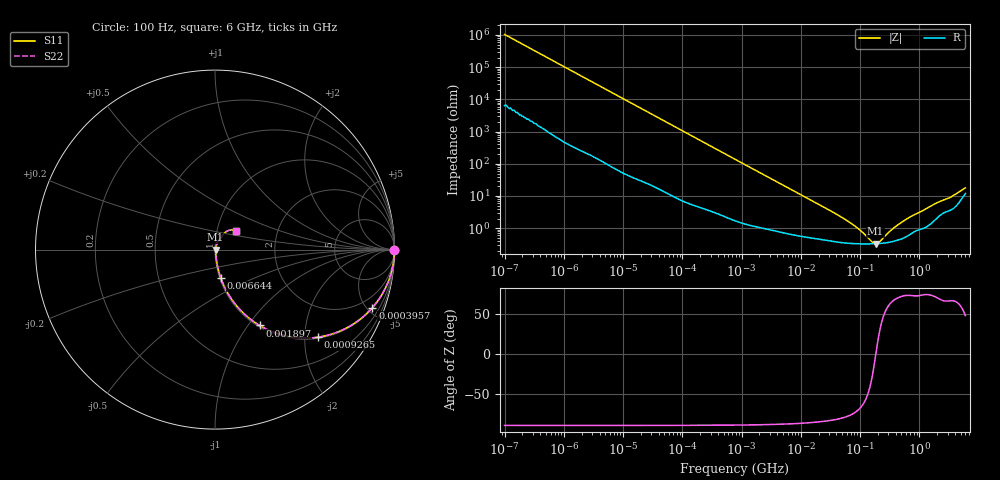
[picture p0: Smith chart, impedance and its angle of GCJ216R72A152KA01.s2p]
!Murata Part Number: GCJ216R72A152KA01
!These Parameters are Measured in Series Mode Connection
!Data Generated on Mar 13, 2026
!  o--ll--o
!Port1  Port2
!  o------o
!Operation Temp=25[degC], DC Bias Voltage=0[V]
!Freq. Start=100[Hz] Stop=6[GHz] 401[Steps]
# Hz S RI R 50
!Freq.(Hz) S11(Real) S11(Imag) S21(Real) S21(Imag) S12(Real) S12(Imag) S22(Real) S22(Imag)
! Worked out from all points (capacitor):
!   401 points, 100 Hz to 6 GHz, reference 50 ohm
!   read as one part in series: C = 1.53 nF near 109 Hz
!   lowest |Z| = 330 mohm at 182.6 MHz (marker M1)
!   series resonance near 184.9 MHz, so ESL is about 480 pH
!   S11 on the Smith chart (normalised r, x): 100 Hz: open; 395.7 kHz: 1.06, -5.41; 926.5 kHz: 1.03, -2.32; 1.897 MHz: 1.02, -1.14; 6.644 MHz: 1.01, -0.33; 6 GHz: 1.24, +0.26
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100  1 -9.62e-05  6e-07 9.62e-05  6e-07 9.62e-05  1 -9.62e-05
2008  1 -0.00191  1.27e-05 0.00191  1.27e-05 0.00191  1 -0.00191
40335  0.9983 -0.038  0.00168 0.038  0.00168 0.038  0.9983 -0.038
141303  0.9818 -0.1303  0.0182 0.1303  0.0182 0.1303  0.9818 -0.1303
395726  0.8771 -0.3233  0.1229 0.3233  0.1229 0.3233  0.8771 -0.3233
774597  0.6559 -0.469  0.3441 0.469  0.3441 0.469  0.6559 -0.469
926525  0.5727 -0.4882  0.4273 0.4882  0.4273 0.4882  0.5727 -0.4882
1896632  0.2486 -0.4229  0.7514 0.4229  0.7514 0.4229  0.2486 -0.4229
3245845  0.1065 -0.2958  0.8935 0.2958  0.8935 0.2958  0.1065 -0.2958
6644369  0.0322 -0.1581  0.9678 0.1581  0.9678 0.1581  0.0322 -0.1581
1.555665e7  0.0098 -0.0697  0.9902 0.0697  0.9902 0.0697  0.0098 -0.0697
6.518806e7  0.00361 -0.0152  0.9964 0.0152  0.9964 0.0152  0.00361 -0.0152
1.020051e8  0.00331 -0.00775  0.9967 0.00775  0.9967 0.00775  0.00331 -0.00775
1.596157e8  0.00326 -0.00182  0.9967 0.00182  0.9967 0.00182  0.00326 -0.00182
1.825626e8  0.00329 -0.000153  0.9967 0.000153  0.9967 0.000153  0.00329 -0.000153
2.183701e8  0.00336 0.00207  0.9966 -0.00207  0.9966 -0.00207  0.00336 0.00207
3.124326e8  0.00369 0.0068  0.9963 -0.0068  0.9963 -0.0068  0.00369 0.0068
4.470121e8  0.00448 0.0123  0.9955 -0.0123  0.9955 -0.0123  0.00448 0.0123
7.31507e8  0.00722 0.0221  0.9928 -0.0221  0.9928 -0.0221  0.00722 0.0221
1.95892e9  0.0228 0.0552  0.9772 -0.0552  0.9772 -0.0552  0.0228 0.0552
3.505958e9  0.0432 0.081  0.9568 -0.081  0.9568 -0.081  0.0432 0.081
6e9  0.1187 0.104  0.8813 -0.104  0.8813 -0.104  0.1187 0.104
